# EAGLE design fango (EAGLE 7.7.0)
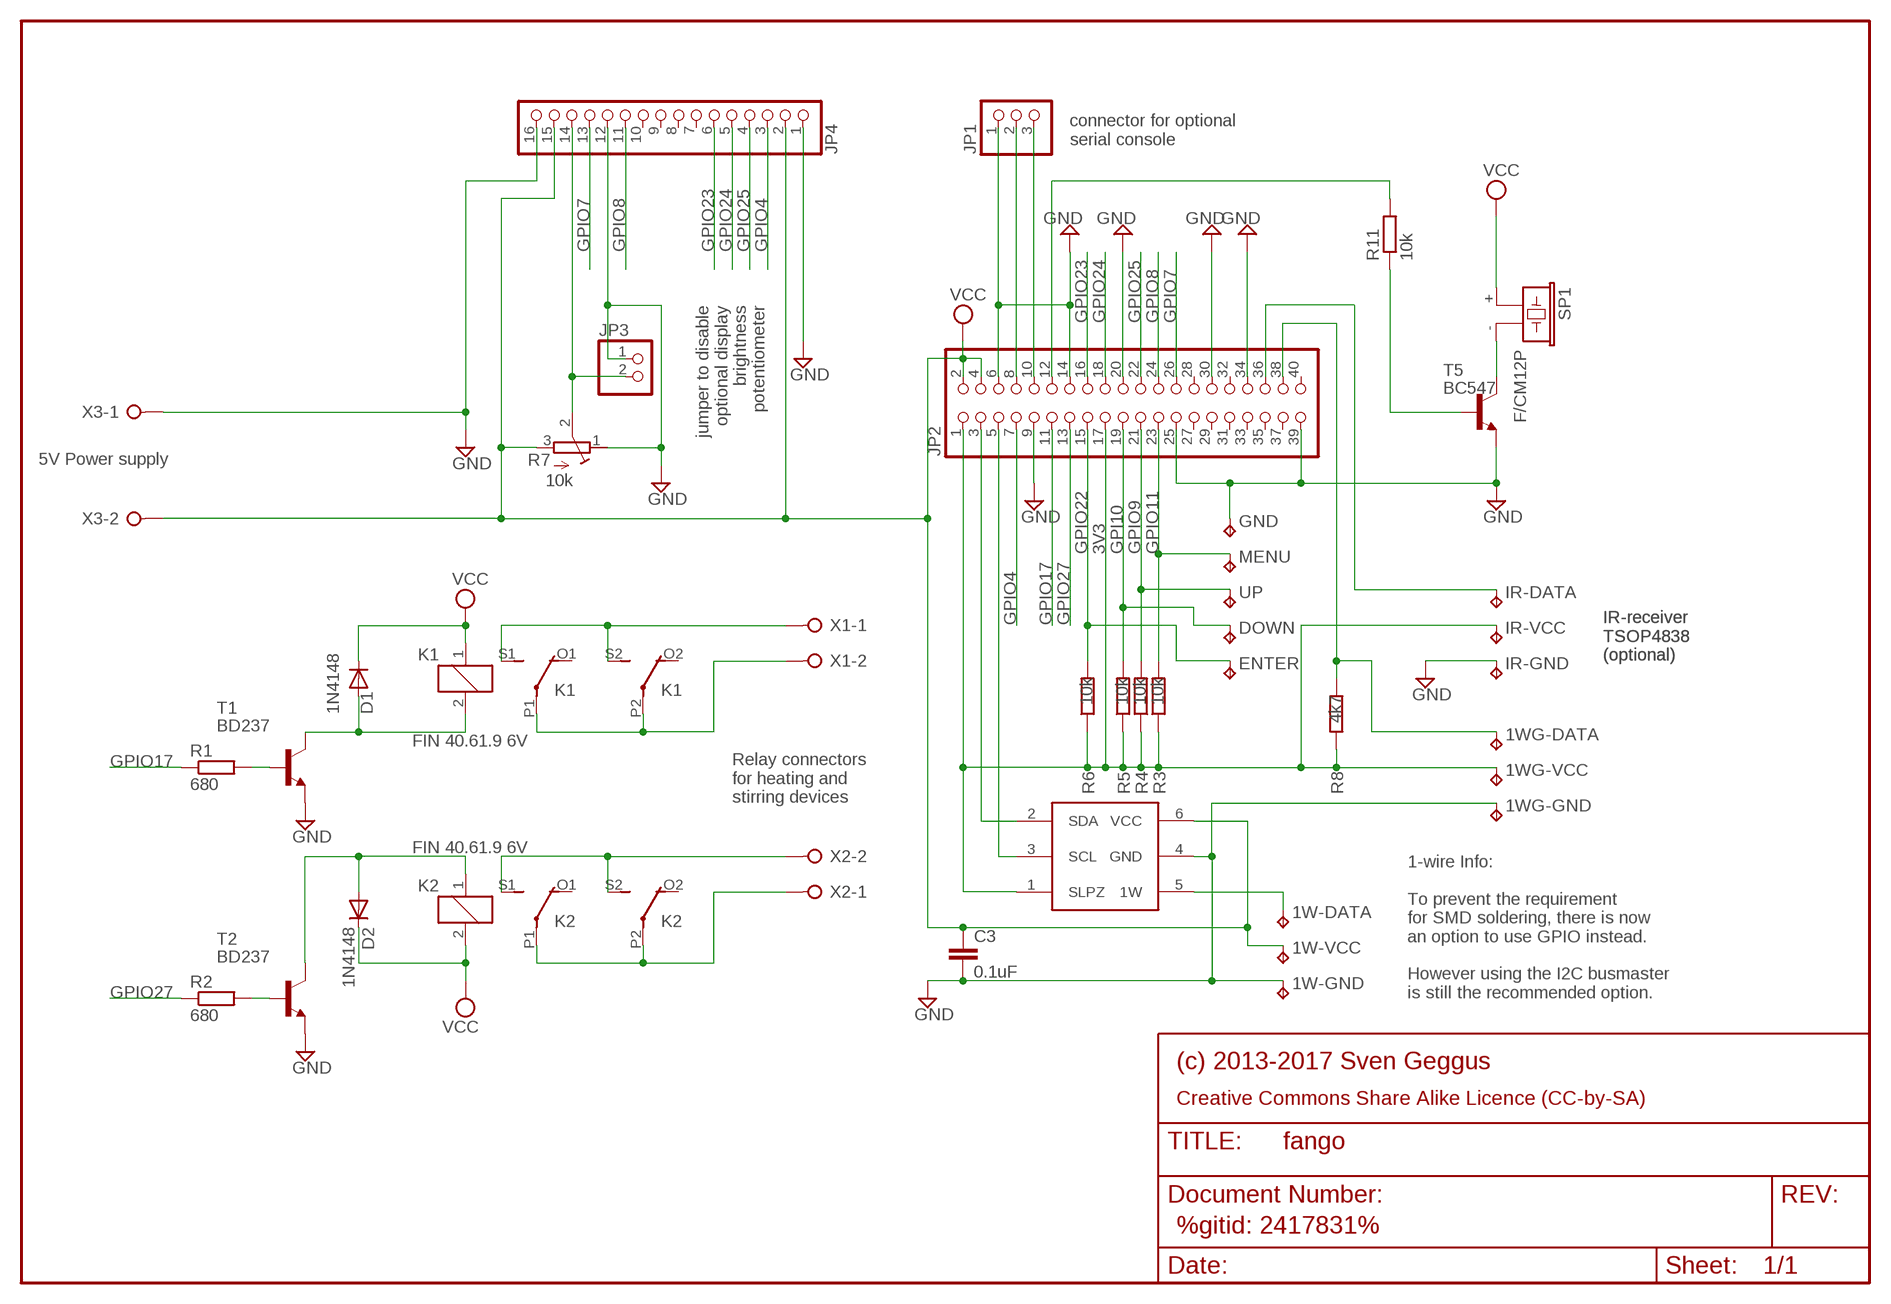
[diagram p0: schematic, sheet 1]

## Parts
1W-DATA  TPPAD1-13  [P1-13]
1W-GND  TPPAD1-13  [P1-13]
1W-VCC  TPPAD1-13  [P1-13]
1WG-DATA  TPPAD1-13  [P1-13]
1WG-GND  TPPAD1-13  [P1-13]
1WG-VCC  TPPAD1-13  [P1-13]
C3  0.1uF  C-EU025-024X044  [C025-024X044]
D1  1N4148  [DO35-10]
D2  1N4148  [DO35-10]
DOWN  TPPAD1-13  [P1-13]
ENTER  TPPAD1-13  [P1-13]
GND  TPPAD1-13  [P1-13]
IC3  DS2483  [TSOT23]
IR-DATA  TPPAD1-13  [P1-13]
IR-GND  TPPAD1-13  [P1-13]
IR-VCC  TPPAD1-13  [P1-13]
JP1  PINHD-1X3  [1X03]
JP2  PINHD-2X20  [2X20]
JP3  PINHD-1X2  [1X02]
JP4  PINHD-1X16  [1X16]
K1  FIN 40.61.9 6V  4052  [F4052]
K2  FIN 40.61.9 6V  4052  [F4052]
MENU  TPPAD1-13  [P1-13]
R1  680  R-EU_0207/10  [0207/10]
R2  680  R-EU_0207/10  [0207/10]
R3  10k  R-EU_0207/10  [0207/10]
R4  10k  R-EU_0207/10  [0207/10]
R5  10k  R-EU_0207/10  [0207/10]
R6  10k  R-EU_0207/10  [0207/10]
R7  10k  R-TRIMM43P  [RTRIM43P]
R8  4k7  R-EU_0207/10  [0207/10]
R11  10k  R-EU_0207/10  [0207/10]
SP1  F/CM12P  [F/CM12P]
T1  BD237  [TO126V]
T2  BD237  [TO126V]
T5  BC547  [TO92]
UP  TPPAD1-13  [P1-13]
X1  W237-02P  [W237-132]
X2  W237-02P  [W237-132]
X3  W237-02P  [W237-132]

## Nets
3V3: 1WG-VCC.TP IC3.1(SLPZ) IR-VCC.TP JP2.1 JP2.17 R3.1 R4.1 R5.1 R6.1 R8.1
GND: 1W-GND.TP 1WG-GND.TP C3.2 GND.TP IC3.4(GND) IR-GND.TP JP1.1 JP2.6 JP2.9 JP2.14 JP2.20 JP2.25 JP2.30 JP2.34 JP2.39 JP3.1 JP4.1 JP4.12 JP4.16 R7.1(E) T1.1(E) T2.1(E) T5.1(E) X3.1
GPI10: DOWN.TP JP2.19 R5.2
GPIO4: JP2.7 JP4.3
GPIO7: JP2.26 JP4.13
GPIO8: JP2.24 JP4.11
GPIO9: JP2.21 R4.2 UP.TP
GPIO11: JP2.23 MENU.TP R3.2
GPIO17: JP2.11 R1.1
GPIO22: ENTER.TP JP2.15 R6.2
GPIO23: JP2.16 JP4.6
GPIO24: JP2.18 JP4.5
GPIO25: JP2.22 JP4.4
GPIO27: JP2.13 R2.1
IR-DATA: IR-DATA.TP JP2.36
N$1: K1.P1(2:P) K1.P2(3:P) X1.2
N$2: R1.2 T1.3(B)
N$4: D2.A K2.1 T2.2(C)
N$5: JP2.12 R11.2
N$6: R11.1 T5.2(B)
N$7: R2.2 T2.3(B)
N$8: K2.P1(2:P) K2.P2(3:P) X2.1
N$9: K1.S1(2:S) K1.S2(3:S) X1.1
N$10: K2.S1(2:S) K2.S2(3:S) X2.2
N$12: JP3.2 JP4.14 R7.2(S)
N$14: SP1.- T5.3(C)
N$16: D1.A K1.2 T1.2(C)
OW: 1W-DATA.TP IC3.5(1W)
OW_SOFT: 1WG-DATA.TP JP2.38 R8.2
OWSCL: IC3.3(SCL) JP2.5
OWSDA: IC3.2(SDA) JP2.3
RXD: JP1.3 JP2.10
TXD: JP1.2 JP2.8
VCC: 1W-VCC.TP C3.1 D1.C D2.C IC3.6(VCC) JP2.2 JP2.4 JP4.2 JP4.15 K1.1 K2.2 R7.3(A) SP1.+ X3.2
Unconnected: JP2.27 JP2.28 JP2.29 JP2.31 JP2.32 JP2.33 JP2.35 JP2.37 JP2.40 JP4.7 JP4.8 JP4.9 JP4.10 K1.O1(2:O) K1.O2(3:O) K2.O1(2:O) K2.O2(3:O)

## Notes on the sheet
- connector for optional
  serial console
- jumper to disable
  optional display
  brightness
  potentiometer
- 5V Power supply
- IR-receiver
  TSOP4838
  (optional)
- IR-receiver
  TSOP4838
  (optional)
- Relay connectors
  for heating and
  stirring devices
- 1-wire Info:
  
  To prevent the requirement
  for SMD soldering, there is now
  an option to use GPIO instead.
  
  However using the I2C busmaster
  is still the recommended option.
- (c) 2013-2017 Sven Geggus
- Creative Commons Share Alike Licence (CC-by-SA)
- %gitid: 2417831%

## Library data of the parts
1W-DATA 1W-GND 1W-VCC 1WG-DATA 1WG-GND 1WG-VCC DOWN ENTER GND IR-DATA IR-GND IR-VCC MENU UP = testpad:TP: Test pad
C3 = rcl:C-EU: CAPACITOR, European symbol
D1 D2 = diode:1N4148: DIODE
IC3 = ds2483:DS2483: Single-Channel 1-Wire Master with Adjustable Timing and Sleep Mode
JP1 = pinhead:PINHD-1X3: PIN HEADER
JP2 = pinhead:PINHD-2X20: PIN HEADER
JP3 = pinhead:PINHD-1X2: PIN HEADER
JP4 = pinhead:PINHD-1X16: PIN HEADER
K1 K2 = relay:4052: RELAY 2 x switch, Finder
R1-R6 R8 R11 = resistor:R-EU_: RESISTOR, European symbol
R7 = rcl:R-TRIMM: Trimm resistor
SP1 = buzzer:F/CM12P: BUZZER; OC_FARNELL: unknown; OC_NEWARK: unknown
T1 T2 = sven-misc:BD237: NPN Transistor
T5 = transistor:BC547: NPN TRANSISTOR
X1-X3 = con-wago-508:W237-02P: WAGO SREW CLAMP; OC_FARNELL: unknown; OC_NEWARK: unknown

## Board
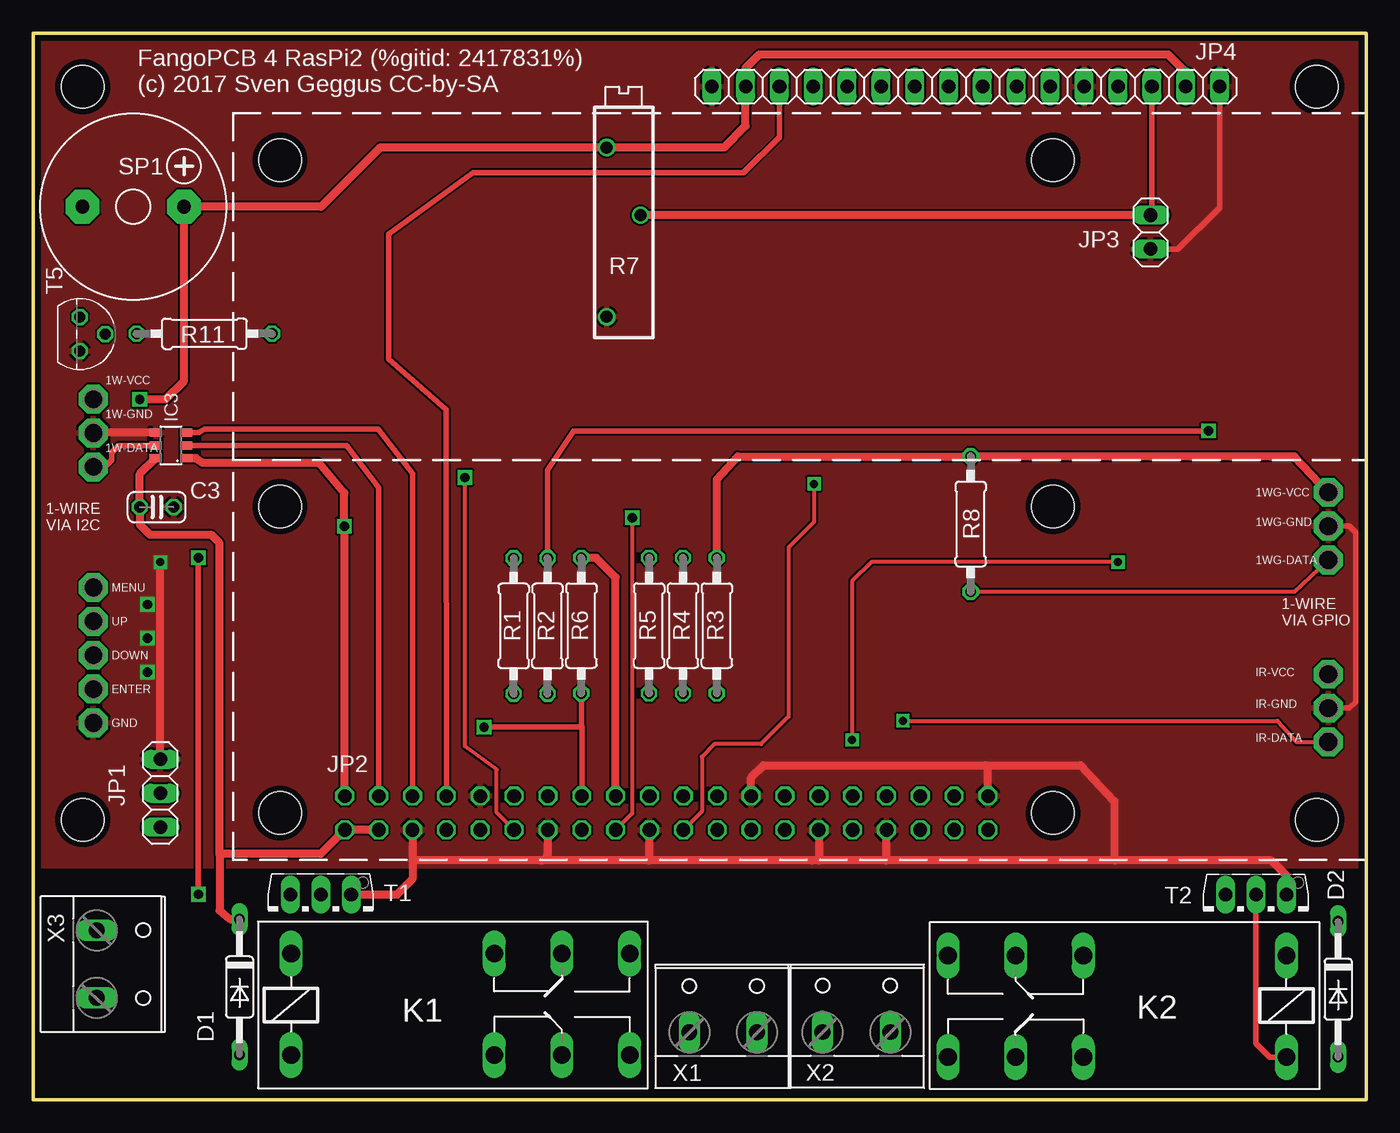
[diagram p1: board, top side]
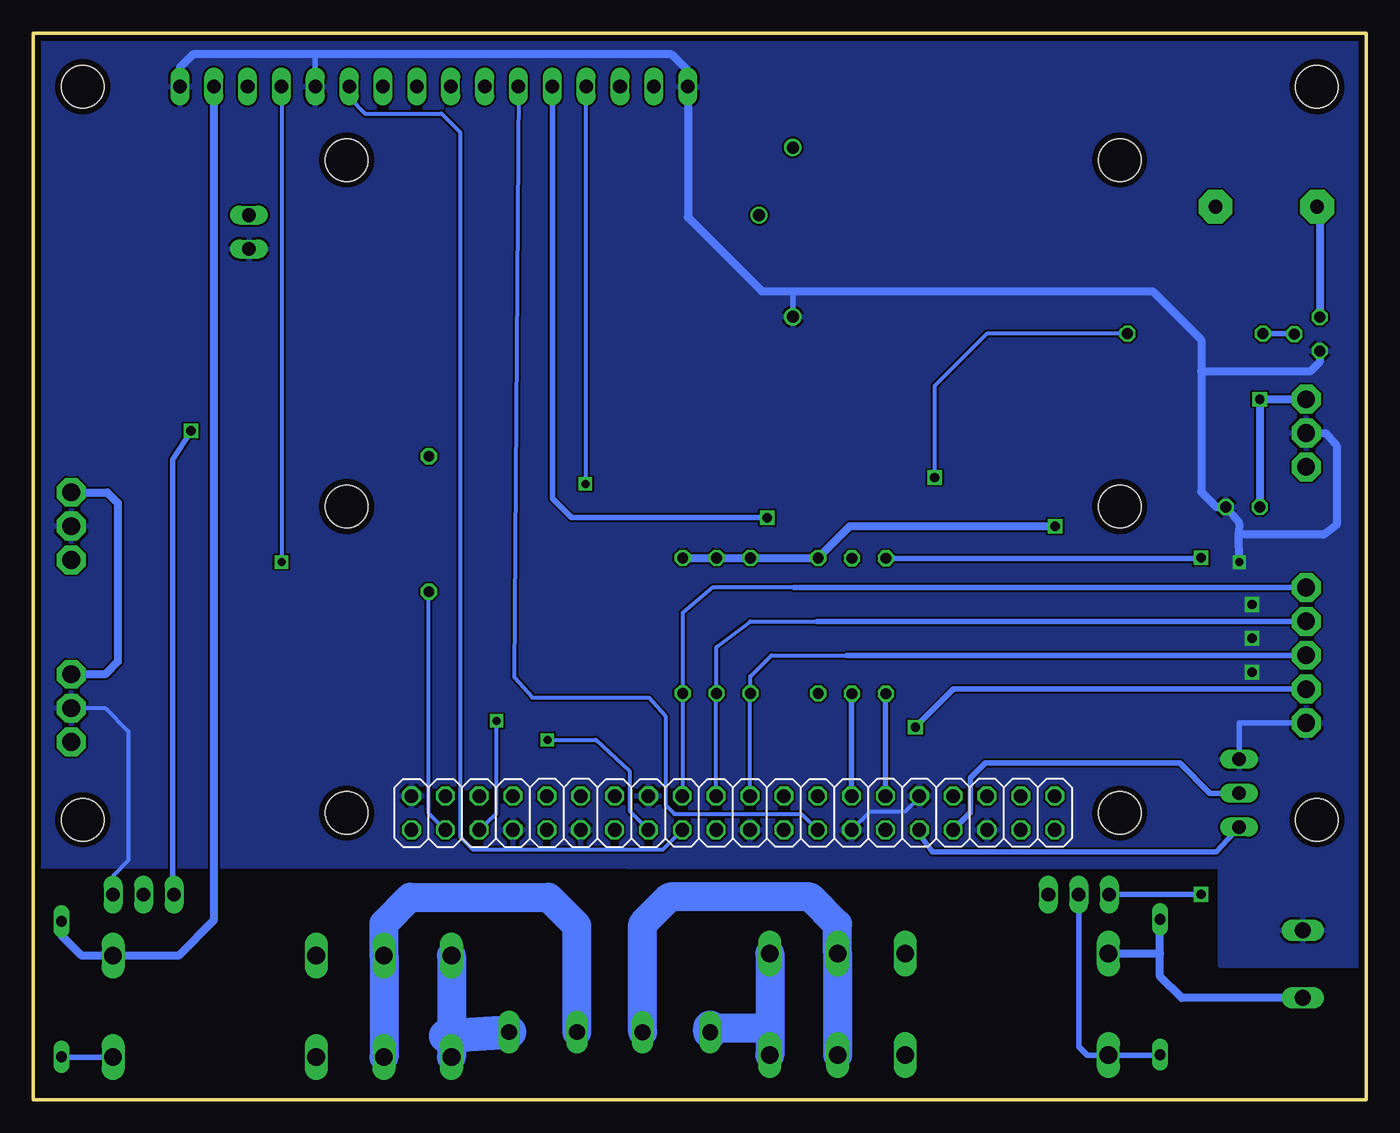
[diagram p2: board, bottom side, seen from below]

Size 100 x 80 mm. Coordinates in mm from the lower left corner, seen from the top.
Outline: 0,0 100,0 100,80 0,80 0,0
Copper layers (1*16): Top 0.018mm / dielectric 1.55mm / Bottom 0.018mm
Design rules "eC-STANDARD_pool-2-layer ": minimum track width 0.15mm, minimum drill 0.25mm, track to track 0.15mm, track to pad 0.15mm, pad to pad 0.15mm, via to via 0.15mm, smd to smd 0.15mm, copper to edge 0.45mm, drill to drill 0.3mm, minimum pad ring 0.2mm, minimum via ring 0.2mm, stop-mask expansion 0.1mm, vias tented up to drill 0mil, thermal gap 0.2mm
Holes 3.2 mm at 76.5,21.5 18.5,21.5 96.3,21 96.3,76 3.7,76 3.7,21 76.5,70.5 18.5,70.5 18.5,44.5 76.5,44.5

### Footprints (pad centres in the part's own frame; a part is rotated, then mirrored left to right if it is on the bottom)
P1-13 = drill 1.321 pad 2.159 octagon: TP 0,0
C025-024X044 = drill 0.813 octagon: 1 -1.27,0; 2 1.27,0
DO35-10 = drill 0.813 long: A 5.08,0; C -5.08,0
TSOT23 = smd 0.6 x 0.9: 1 -0.95,-1.15; 2 0,-1.15; 3 0.95,-1.15; 4 0.95,1.15; 5 0,1.15; 6 -0.95,1.15
1X03 = drill 1.016 long: 1 -2.54,0; 2 0,0; 3 2.54,0
2X20 = drill 1.016 octagon: 1 -24.13,-1.27; 2 -24.13,1.27; 3 -21.59,-1.27; 4 -21.59,1.27; 5 -19.05,-1.27; 6 -19.05,1.27; 7 -16.51,-1.27; 8 -16.51,1.27; 9 -13.97,-1.27; 10 -13.97,1.27; 11 -11.43,-1.27; 12 -11.43,1.27; 13 -8.89,-1.27; 14 -8.89,1.27; 15 -6.35,-1.27; 16 -6.35,1.27; 17 -3.81,-1.27; 18 -3.81,1.27; 19 -1.27,-1.27; 20 -1.27,1.27; 21 1.27,-1.27; 22 1.27,1.27; 23 3.81,-1.27; 24 3.81,1.27; 25 6.35,-1.27; 26 6.35,1.27; 27 8.89,-1.27; 28 8.89,1.27; 29 11.43,-1.27; 30 11.43,1.27; 31 13.97,-1.27; 32 13.97,1.27; 33 16.51,-1.27; 34 16.51,1.27; 35 19.05,-1.27; 36 19.05,1.27; 37 21.59,-1.27; 38 21.59,1.27; 39 24.13,-1.27; 40 24.13,1.27
1X02 = drill 1.016 long: 1 -1.27,0; 2 1.27,0
1X16 = drill 1.016 long: 1 -19.05,0; 2 -16.51,0; 3 -13.97,0; 4 -11.43,0; 5 -8.89,0; 6 -6.35,0; 7 -3.81,0; 8 -1.27,0; 9 1.27,0; 10 3.81,0; 11 6.35,0; 12 8.89,0; 13 11.43,0; 14 13.97,0; 15 16.51,0; 16 19.05,0
F4052 = drill 1.321 long: 1 -3.81,3.81; 2 -3.81,-3.81; O1 11.43,-3.81; O2 11.43,3.81; P1 16.51,-3.81; P2 16.51,3.81; S1 21.59,-3.81; S2 21.59,3.81
0207/10 = drill 0.813 octagon: 1 -5.08,0; 2 5.08,0
RTRIM43P = drill 0.9: 1 -7.62,1.27; 2 0,-1.27; 3 5.08,1.27
F/CM12P = drill 1.016 pad 2.54 octagon: + 3.81,0; - -3.81,0
TO126V = drill 1.016 long: 1 -2.286,-1.27; 2 0,-1.27; 3 2.286,-1.27
TO92 = drill 0.813 octagon: 1 1.27,0; 2 0,1.905; 3 -1.27,0
W237-132 = drill 1.194 long: 1 -2.54,-0.635; 2 2.54,-0.635

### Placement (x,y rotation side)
1W-DATA  4.5,47.47 0 top
1W-GND  4.5,50.01 0 top
1W-VCC  4.5,52.55 0 top
1WG-DATA  97.16,40.48 0 top
1WG-GND  97.16,43.02 0 top
1WG-VCC  97.16,45.56 0 top
C3  9.26,44.45 0 top
D1  15.47,8.45 270 top
D2  97.89,8.29 270 top
DOWN  4.5,33.34 0 top
ENTER  4.5,30.8 0 top
GND  4.5,28.26 0 top
IC3  10.32,49.09 90 top
IR-DATA  97.16,26.83 0 top
IR-GND  97.16,29.37 0 top
IR-VCC  97.16,31.91 0 top
JP1  9.53,22.99 270 top
JP2  47.5,21.5 180 bottom
JP3  83.82,65.09 90 top
JP4  69.95,76 0 top
K1  23.15,7.14 0 top
K2  90.21,6.99 180 top
MENU  4.5,38.42 0 top
R1  36.04,35.53 90 top
R2  38.58,35.53 90 top
R3  51.28,35.56 270 top
R4  48.74,35.56 270 top
R5  46.2,35.56 270 top
R6  41.12,35.56 270 top
R7  44.29,66.36 90 top
R8  70.33,43.18 270 top
R11  12.83,57.47 0 top
SP1  7.49,66.99 0 top
T1  21.56,14.12 180 top
T2  91.73,14.11 180 top
T5  3.49,57.44 270 top
UP  4.5,35.88 0 top
X1  51.75,5.68 0 top
X2  61.75,5.7 0 top
X3  5.4,10.16 270 top

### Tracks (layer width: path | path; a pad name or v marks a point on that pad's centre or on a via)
3V3  (via drill 0.7)
  Top 0.61: JP2.17 43.69,39.18 42.23,40.64 R6.1 | IC3.1 12.19,48.13 12.7,47.78 21.39,47.78 23.34,45.52 v23.34,43.02 23.37,42.99 JP2.1 | R3.1 51.28,46.51 52.86,48.26 R8.1 94.61,48.26 1WG-VCC.TP
  Bottom 0.61: R3.1 R4.1 R5.1 R6.1 38.73,43.02 v23.34,43.02 | 1WG-VCC.TP 94.46,45.56 93.66,44.77 93.66,32.86 94.61,31.91 IR-VCC.TP
GND  (via drill 0.6, 0.7)
  Top 0.305: 71.63,24.89 71.44,25.08
  Top 0.406: IR-GND.TP 98.74,29.37 99.22,29.84 99.22,42.55 98.74,43.02 1WG-GND.TP | JP3.1 85.88,63.82 89,66.93 JP4.16 | 58.93,17.94 58.42,17.94
  Top 0.61: IC3.4 4,50.03 1W-GND.TP | JP2.6 28.45,17.94 | 28.45,17.94 28.45,16.54 27.3,15.39 T1.1 | 81.12,17.94 92.88,17.94 94.01,16.8 T2.1 | 81.12,17.94 63.98,17.94 | 63.98,17.94 58.42,17.94 46.2,17.94 | 46.2,17.94 38.1,17.94 | 38.1,17.94 28.45,17.94 | 46.2,20 46.2,17.94 | 38.58,20.32 38.58,18.41 arc-90 38.1,17.94 | 81.12,17.94 81.12,22.38 78.58,25.08 71.44,25.08 54.77,25.08 53.85,24.16 JP2.25 | JP1.1 v9.53,40.32 | JP2.30 58.93,17.94 | 63.98,20.2 63.98,17.94 | JP2.39 71.63,24.89
  Bottom 0.305: JP2.9 33.53,22.67 34.61,21.59 37.25,21.59 JP2.14 | IR-GND.TP 94.61,29.37 92.87,27.62 92.87,17.95 93.98,16.83 93.98,15.4 T2.1
  Bottom 0.406: 45.34,60.64 43.02,60.64 R7.1 | 88.02,78.42 78.84,78.42 JP4.12 | JP1.1 9.53,28.26 GND.TP
  Bottom 0.61: JP4.16 89,77.45 88.02,78.42 52.13,78.42 50.9,77.19 JP4.1 50.9,66.2 45.34,60.64 16.01,60.64 12.38,57.02 12.38,54.63 | 12.38,54.63 12.38,45.59 11.24,44.45 C3.2 9.53,43.24 9.55,42.53 | 9.55,42.53 9.56,42.17 | T5.1 3.49,55.34 4.2,54.63 12.38,54.63 | 1W-GND.TP 3.04,50.01 2.18,48.98 2.18,43.19 3.18,42.39 9.55,42.39 | v9.53,40.32 9.55,42.39 | 9.55,42.39 9.55,42.53
  other vias: 8.57,37.15 8.57,34.61 8.57,32.07
  pour Bottom: 0,10.06 0,80 100,80 100,17.52 10.95,17.46 10.95,10.06
  pour Top: 0,17.52 0,80 100,80 100,17.52
GPI10
  Bottom 0.305: JP2.19 46.23,30.45 R5.2 46.2,31.75 44.61,33.34 38.94,33.34
  Bottom 0.406: DOWN.TP 38.94,33.34
GPIO4
  Top 0.406: JP4.3 55.98,72.22 53.3,69.53 33,69.53 26.67,64.95 26.67,55.56 30.96,51.75 JP2.7
GPIO7  (via drill 0.6)
  Top 0.305: v81.38,40.32 62.87,40.32 61.44,38.89 v61.44,26.99
  Bottom 0.305: JP4.13 v81.38,40.32 | JP2.26 55.24,21.62 55.24,24.61 57.78,26.99 v61.44,26.99
GPIO8
  Bottom 0.305: JP2.24 52.81,18.73 66.99,18.73 67.94,19.68 67.94,72.55 69.37,73.98 75.09,73.98 76.3,75.19 JP4.11
GPIO9
  Bottom 0.305: JP2.21 48.77,30.45 R4.2 48.74,33.97 46.2,35.88 41.19,35.88
  Bottom 0.406: UP.TP 41.19,35.88
GPIO11
  Bottom 0.305: 42.95,38.42 49.05,38.42 51.28,36.51 R3.2 51.28,22.8 JP2.23
  Bottom 0.406: MENU.TP 42.95,38.42
GPIO17
  Bottom 0.406: JP2.11 36.07,30.45 R1.1
GPIO22  (via drill 0.7)
  Top 0.406: JP2.15 41.15,27.94 41.12,27.94 | 41.12,27.94 v33.81,27.94 | R6.2 41.12,27.94
  Bottom 0.406: ENTER.TP 30.96,30.8 v33.81,27.94
GPIO23
  Bottom 0.305: JP4.6 63.92,31.69 62.55,30.16 53.82,30.16 52.55,28.73 52.55,22.07 51.91,21.43 42.35,21.43 JP2.16
GPIO24  (via drill 0.7)
  Top 0.305: v44.93,43.66 44.93,21.47 JP2.18
  Bottom 0.406: v44.93,43.66 59.63,43.66 61.06,45.08 JP4.5
GPIO25  (via drill 0.6)
  Top 0.305: v58.58,46.2 58.58,43.34 56.67,41.43 56.67,28.73 54.61,26.67 51.12,26.67 50.16,25.72 50.16,21.62 JP2.22
  Bottom 0.305: JP4.4 arc-90 58.58,75.94 v58.58,46.2
GPIO27
  Bottom 0.406: JP2.13 38.61,30.45 R2.1
IR-DATA  (via drill 0.6)
  Top 0.305: IR-DATA.TP 94.77,26.83 93.34,28.42 v65.25,28.42
  Bottom 0.305: v65.25,28.42 65.25,21.47 JP2.36
N$1
  Bottom 2.184: K1.P1 K1.P2 39.66,13.16 41.7,15.2 52.26,15.2 54.29,13.17 X1.2
N$2  (via drill 0.7)
  Top 0.406: v12.38,40.64 v12.38,15.39
  Bottom 0.406: v12.38,15.39 T1.3 | R1.2 12.41,40.61 v12.38,40.64
N$4
  Top 0.406: T2.2 91.73,4.21 92.76,3.18 K2.1
  Bottom 0.406: K2.1 97.89,3.18 D2.A
N$5  (via drill 0.7)
  Top 0.305: JP2.12 34.77,21.53 34.77,24.77 32.38,26.51 v32.38,46.67
  Bottom 0.305: R11.2 28.47,57.47 32.38,53.55 v32.38,46.67
N$6
  Bottom 0.406: R11.1 5.4,57.47 T5.2
N$7  (via drill 0.7)
  Top 0.406: v88.17,50.16 40.55,50.16 38.58,47.24 R2.2
  Bottom 0.406: T2.3 89.53,15.38 89.53,48.01 v88.17,50.16
N$8
  Bottom 2.184: K2.P2 K2.P1 73.7,13.2 71.72,15.18 61.34,15.18 59.21,13.05 X2.1
N$9
  Bottom 2.184: K1.S2 44.74,5.4 | 44.74,5.4 K1.S1 | 49.21,5.4 44.74,5.4
  Bottom 2.54: X1.1 49.21,5.4
N$10
  Bottom 2.184: K2.S1 68.62,4.76 | 68.62,4.76 K2.S2 | 69.06,4.76 68.62,4.76
  Bottom 2.54: X2.2 69.06,4.76
N$12
  Top 0.406: JP3.2 83.92,66.36 JP4.14
  Top 0.61: JP3.2 R7.2
N$14
  Bottom 0.406: SP1.- 3.49,66.99
  Bottom 0.61: 3.49,66.99 T5.3
N$16
  Bottom 0.406: T1.2 21.56,3.97 20.92,3.33 K1.2 15.47,3.33 D1.A
OW
  Top 0.406: IC3.5 6.41,49.09 5.87,48.55 5.87,47.97 5.37,47.47 1W-DATA.TP
OW_SOFT
  Top 0.305: R8.2 94.61,38.1 1WG-DATA.TP
  Bottom 0.305: JP2.38 70.33,21.47 R8.2
OWSCL
  Top 0.406: JP2.5 28.45,46.96 25.88,50.32 12.86,50.32 12.41,50.03 IC3.3
OWSDA
  Top 0.406: IC3.2 23.52,49.09 25.91,45.91 JP2.3
RXD
  Bottom 0.406: JP2.10 33.53,19.88 32.54,18.57 11.24,18.57 JP1.3
TXD
  Bottom 0.406: JP2.8 29.69,21.53 29.69,24.13 28.57,25.24 13.97,25.24 11.72,22.99 JP1.2
VCC  (via drill 0.7)
  Top 0.406: JP4.2 53.5,76 | SP1.+ 11.27,66.99
  Top 0.61: JP4.15 86.46,77.09 85.13,78.42 54.46,78.42 53.44,77.4 JP4.2 53.44,73.06 51.82,71.44 R7.3 26.04,71.44 21.59,66.99 SP1.+ 11.3,53.92 9.93,52.55 v7.99,52.55 | D1.C 14.78,13.53 13.97,14.18 13.97,18.41 | JP2.4 JP2.2 21.55,18.41 13.97,18.41 | 13.97,18.41 13.97,41.75 13.34,42.39 8.73,42.39 7.99,43.13 C3.1 7.99,46.95 IC3.6
  Bottom 0.406: 15.47,10.96 D1.C
  Bottom 0.61: 1W-VCC.TP v7.99,52.55 C3.1 | D2.C 97.89,12.34 96.35,10.8 K2.2 89.11,10.8 86.46,13.45 JP4.15 | X3.2 13.85,7.62 15.47,9.24 D1.C | K1.1 15.47,10.96

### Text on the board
tNames: FangoPCB 4 RasPi2 (%gitid: 2417831%) / (c) 2017 Sven Geggus CC-by-SA | 1-WIRE / VIA I2C | 1-WIRE / VIA GPIO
